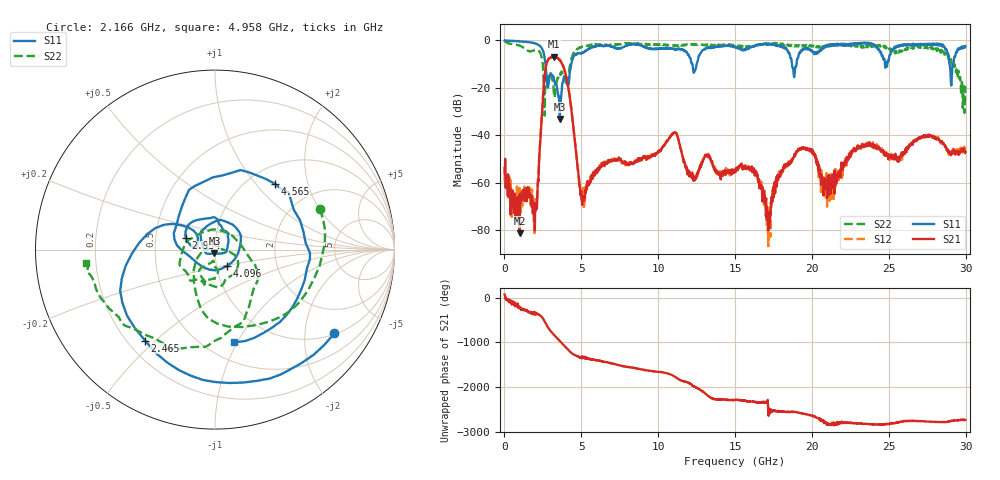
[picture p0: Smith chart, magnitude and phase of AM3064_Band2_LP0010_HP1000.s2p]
# Hz S DB R 50.0
!freq dBS11 angS11 dBS21 angS21 dBS12 angS12 dBS22 angS22
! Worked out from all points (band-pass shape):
!   1600 points, 10 MHz to 29.98 GHz, reference 50 ohm
!   highest |S21| = -6.79 dB at 3.215 GHz (marker M1); lowest = -81.3 dB at 984.7 MHz (marker M2)
!   |S21| within 3 dB of the highest: 2.739 GHz to 3.745 GHz (1.007 GHz wide, 31 % of centre)
!   lowest |S11| = -33.2 dB at 3.609 GHz (marker M3), VSWR 1.04, Z = 49.6 - j2.15 ohm
!   |S11| at or under -10 dB: 2.671 GHz to 4.346 GHz (1.674 GHz wide, 47.7 % of centre); 12.23 GHz to 12.5 GHz (272.2 MHz wide, 2.2 % of centre); 18.7 GHz to 19 GHz (297.7 MHz wide, 1.58 % of centre)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
!   |S22| runs from -31.7 to -0.2 dB; largest |S21 - S12| = 0.017
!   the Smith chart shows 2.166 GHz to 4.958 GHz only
!   S11 on the Smith chart (normalised r, x): 2.166 GHz: 1.03, -2.83; 2.465 GHz: 0.27, -0.46; 2.934 GHz: 0.71, +0.09; 4.096 GHz: 1.12, -0.21; 4.565 GHz: 1.30, +1.26; 4.958 GHz: 0.68, -0.97
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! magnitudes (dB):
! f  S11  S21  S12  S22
! 10 MHz  0.0  -53.8  -56.5  -0.2
! 984.7 MHz  -0.4  -81.3  -62.2  -2.2
! 2.166 GHz  -1.8  -60.5  -60.7  -4.1
! 2.465 GHz  -3.9  -27.6  -27.5  -8.3
! 2.934 GHz  -15.2  -7.5  -7.5  -13.6
! 3.215 GHz  -16.0  -6.8  -7.0  -22.1
! 3.609 GHz  -33.2  -8.5  -8.3  -14.0
! 4.096 GHz  -19.0  -17.8  -17.5  -18.7
! 4.565 GHz  -6.1  -41.6  -41.4  -4.5
! 4.958 GHz  -5.6  -65.2  -63.2  -2.8
! 5.015 GHz  -5.6  -66.8  -65.2  -2.9
! 10 GHz  -3.5  -46.9  -46.8  -1.8
! 15 GHz  -2.6  -54.7  -55.2  -1.8
! 16.32 GHz  -2.2  -55.3  -55.5  -2.0
! 17.16 GHz  -1.6  -80.2  -86.7  -1.4
! 18.12 GHz  -3.1  -54.9  -55.2  -1.6
! 19.99 GHz  -4.3  -46.9  -47.1  -2.1
! 21.12 GHz  -1.8  -56.7  -64.2  -2.6
! 23.01 GHz  -1.5  -45.3  -45.2  -2.6
! 25 GHz  -8.4  -48.2  -48.1  -3.0
! 28.56 GHz  -2.5  -43.6  -43.7  -4.7
! 29.98 GHz  -2.4  -47.0  -47.3  -19.2
